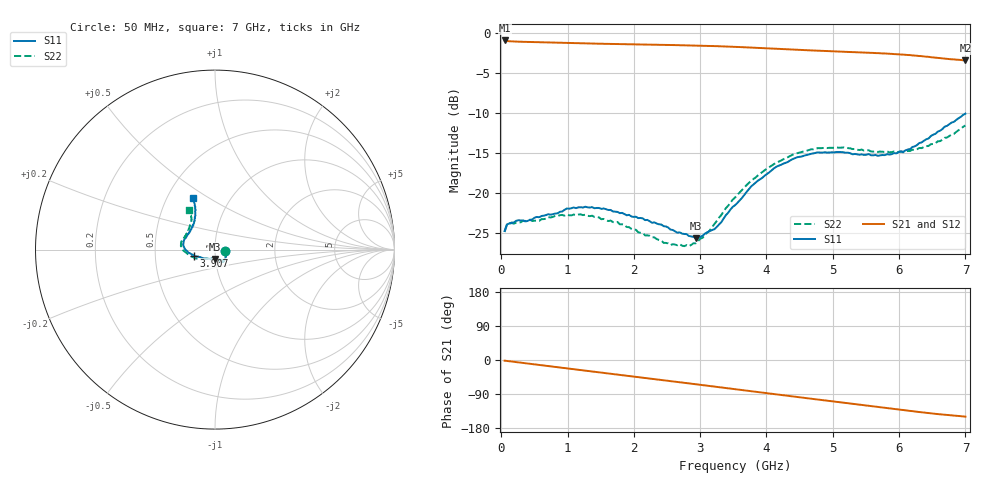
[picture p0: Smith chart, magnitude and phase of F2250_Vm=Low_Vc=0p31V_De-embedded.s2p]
! Integrated Device Technology
! Corporate Headquarters
! 6024 Silver Creek Valley Road
! San Jose, CA 95138  USA
! Phone:  1-408-284-8200
! Toll Free:  1-800-223-1366
! Webpage:  http://www.idt.com/
! Timing and RF Division
! 515 Groton Road, Suite 102
! Westford, MA 01886-6024
! Device:  F2250
! Description: Voltage Variable RF Attenuator
! Frequency:  50.0 -  6000.00 MHz
! Package:  3x3 mm Thin QFN Plastic Package: 16 pin
! Ports:  2 RF, 3 DC
!  Pin  1  = GND
!  Pin  2  = NC
!  Pin  3  = RF1  = Port 1
!  Pin  4  = NC
!  Pin  5  = GND
!  Pin  6  = GND
!  Pin  7  = GND
!  Pin  8  = GND
!  Pin  9  = NC
!  Pin 10  = RF2  = Port 2
!  Pin 11  = NC
!  Pin 12  = GND
!  Pin 13  = GND
!  Pin 14  = VCNTRL
!  Pin 15  = VDD
!  Pin 16  = VMODE
! Vcntrl:  0.310 Volts
! Vmode:  +0.000 Volts
! Vdd:  +3.30  Volts
! Current:  1.114 mA
! Data:  The device was measured on a the F2250 evaluation board which has
!  individual transmission lines to the RF pins.  Data was collected
!  using a calibrated network analyzer.  The evaluation board was
!  de-embedded using a TRL calibration technique.
!  The reference plane is the edge of the package pin.
! Misc:  SN 10
!  Action Tracker AT0258
! Date Measured:  2014-11-26
! Date:  2015-10-15  MJV
! Note:
!  Integrated Device Technology supplies this data as a sample of measured
!  data at the package pin for this product.  Your particular data for this
!  product may vary.
!  Data was taken at 25 degrees C.
!  Integrated Device Technology reserves the right to change this data at anytime.
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# GHz S dB R 50
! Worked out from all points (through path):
!   201 points, 50 MHz to 7 GHz, reference 50 ohm
!   highest |S21| = -0.95 dB at 50 MHz (marker M1); lowest = -3.4 dB at 7 GHz (marker M2)
!   group delay of S21, straight-line fit = 60 ps
!   lowest |S11| = -25.6 dB at 2.934 GHz (marker M3), VSWR 1.11, Z = 49.7 - j5.23 ohm
!   |S11| at or under -10 dB: start of sweep to end of sweep
!   |S22| runs from -26.6 to -11.6 dB; largest |S21 - S12| = 0.00037
!   S11 on the Smith chart (normalised r, x): 50 MHz: 1.12, -0.02; 3.907 GHz: 0.79, -0.05; 7 GHz: 0.67, +0.43
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0.05  -24.69 -9.3  -0.95 -1.8  -0.95 -1.8  -24.82 -9.8
0.08475  -23.88 -9.2  -1.02 -2.5  -1.02 -2.5  -23.95 -9.1
0.15425  -23.66 -11.5  -1.07 -4.0  -1.07 -4.0  -23.72 -10.8
0.57125  -22.98 -29.2  -1.17 -13.1  -1.17 -13.1  -23.44 -29.9
0.884  -22.31 -44.7  -1.24 -19.9  -1.23 -19.9  -22.72 -46.2
1.2315  -21.78 -54.7  -1.31 -27.4  -1.31 -27.4  -22.72 -59.0
1.75275  -22.32 -61.5  -1.40 -38.4  -1.40 -38.4  -23.58 -66.2
2.37825  -23.86 -62.4  -1.49 -51.8  -1.49 -51.8  -25.82 -68.4
2.552  -24.53 -66.4  -1.52 -55.6  -1.52 -55.6  -26.46 -74.0
2.83  -25.33 -81.3  -1.57 -61.7  -1.57 -61.7  -26.59 -92.9
2.93425  -25.61 -90.0  -1.59 -64.0  -1.59 -64.0  -26.24 -101.5
3.21225  -24.49 -119.4  -1.66 -70.2  -1.65 -70.2  -23.86 -127.0
3.525  -21.50 -146.4  -1.75 -77.1  -1.75 -77.1  -20.53 -145.8
3.76825  -19.16 -159.9  -1.84 -82.5  -1.84 -82.5  -18.43 -156.3
3.90725  -18.24 -164.3  -1.90 -85.5  -1.89 -85.5  -17.55 -162.4
4.1505  -16.68 -172.7  -1.99 -90.8  -1.99 -90.8  -16.18 -171.1
4.7065  -15.03 173.0  -2.20 -102.9  -2.20 -102.9  -14.52 175.8
5.15825  -14.89 162.2  -2.36 -112.6  -2.36 -112.6  -14.29 166.6
5.85325  -15.17 139.0  -2.61 -127.5  -2.61 -127.5  -14.90 151.5
6.166  -14.49 128.1  -2.78 -134.3  -2.78 -134.3  -14.72 142.7
6.444  -13.17 119.7  -2.99 -140.1  -2.99 -140.1  -14.11 133.3
7  -10.08 113.3  -3.43 -149.4  -3.43 -149.4  -11.55 123.8
